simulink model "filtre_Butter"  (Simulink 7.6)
settings: Solver=ode15s  StartTime=0.0  StopTime=N  RelTol=1e-3
StopFcn:
  | courbes_butter
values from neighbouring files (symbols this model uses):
  R1 = 1e3    (= 1000)    [filtre_pbande.m]    (also in impedance_quartz.m = 30; Calcul_symbolique_RLC.m = 1)
  R2 = 100e3    (= 100000)    [_startup.m]    (also in filtre_pbande.m = 10000; Calcul_symbolique_RLC.m = 1)
libraries: fl_lib x24, nesl_utility x4, elec_lib x1

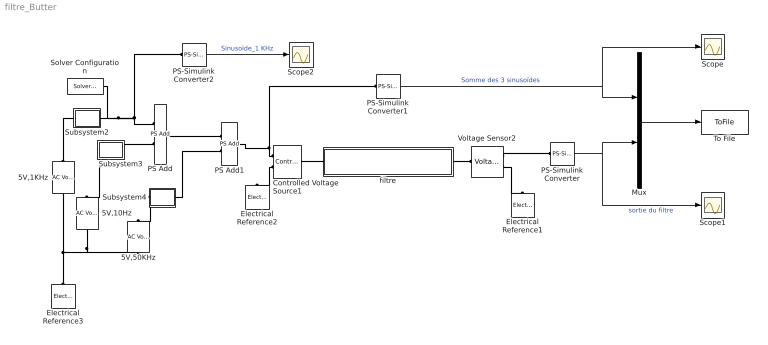
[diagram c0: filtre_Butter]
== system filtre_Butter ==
  5V,10Hz : fl_lib/Electrical/Electrical Sources/AC Voltage Source  DialogController=NetworkEngine.DynNeDlgSource  SystemSampleTime=-1  amp=5 V  shift=0 rad  omega=10 Hz  i_Log=off  v_Log=off  LocalVarNames=|current|voltage|power  LocalVarDescs=|Current (A)|Voltage (V)|Power (W)  LocalVarLogging=[0 0 0]
  5V,1KHz : fl_lib/Electrical/Electrical Sources/AC Voltage Source  DialogController=NetworkEngine.DynNeDlgSource  SystemSampleTime=-1  amp=5 V  shift=0 rad  omega=1 kHz  i_Log=off  v_Log=off  LocalVarNames=|current|voltage|power  LocalVarDescs=|Current (A)|Voltage (V)|Power (W)  LocalVarLogging=[0 0 0]
  5V,50KHz : fl_lib/Electrical/Electrical Sources/AC Voltage Source  DialogController=NetworkEngine.DynNeDlgSource  SystemSampleTime=-1  amp=5 V  shift=0 rad  omega=50 kHz  i_Log=off  v_Log=off  LocalVarNames=|current|voltage|power  LocalVarDescs=|Current (A)|Voltage (V)|Power (W)  LocalVarLogging=[0 0 0]
  Controlled Voltage Source1 : fl_lib/Electrical/Electrical Sources/Controlled Voltage Source  DialogController=NetworkEngine.DynNeDlgSource  SystemSampleTime=-1  i_Log=off  v_Log=off  LocalVarNames=|current|voltage|power  LocalVarDescs=|Current (A)|Voltage (V)|Power (W)  LocalVarLogging=[0 0 0]
  Electrical Reference1 : fl_lib/Electrical/Electrical Elements/Electrical Reference  DialogController=NetworkEngine.DynNeDlgSource  SystemSampleTime=-1  i_Log=off  LocalVarNames=|i  LocalVarDescs=|i  LocalVarLogging=0
  Electrical Reference2 : fl_lib/Electrical/Electrical Elements/Electrical Reference  DialogController=NetworkEngine.DynNeDlgSource  SystemSampleTime=-1  i_Log=off  LocalVarNames=|i  LocalVarDescs=|i  LocalVarLogging=0
  Electrical Reference3 : fl_lib/Electrical/Electrical Elements/Electrical Reference  DialogController=NetworkEngine.DynNeDlgSource  SystemSampleTime=-1  i_Log=off  LocalVarNames=|i  LocalVarDescs=|i  LocalVarLogging=0
  Mux : Mux  Inputs=2
  PS Add : fl_lib/Physical Signals/Functions/PS Add  DialogController=NetworkEngine.DynNeDlgSource  SystemSampleTime=-1  LocalVarLogging=[]
  PS Add1 : fl_lib/Physical Signals/Functions/PS Add  DialogController=NetworkEngine.DynNeDlgSource  SystemSampleTime=-1  LocalVarLogging=[]
  PS-Simulink Converter : nesl_utility/PS-Simulink Converter  DialogController=NetworkEngine.DynNeUtilDlgSource  SystemSampleTime=-1  PhysicalDomain=network_engine_domain  LeftPortType=input  RightPortType=output  SubClassName=ps_output  Unit=1  AffineConversion=off
  PS-Simulink Converter1 : nesl_utility/PS-Simulink Converter  DialogController=NetworkEngine.DynNeUtilDlgSource  SystemSampleTime=-1  PhysicalDomain=network_engine_domain  LeftPortType=input  RightPortType=output  SubClassName=ps_output  Unit=1  AffineConversion=off
  PS-Simulink Converter2 : nesl_utility/PS-Simulink Converter  DialogController=NetworkEngine.DynNeUtilDlgSource  SystemSampleTime=-1  PhysicalDomain=network_engine_domain  LeftPortType=input  RightPortType=output  SubClassName=ps_output  Unit=1  AffineConversion=off
  Scope : Scope
  Scope1 : Scope
  Scope2 : Scope
  Solver Configuration : nesl_utility/Solver Configuration  DialogController=NetworkEngine.DynNeUtilDlgSource  SystemSampleTime=-1  PhysicalDomain=network_engine_domain  LeftPortType=input  RightPortType=generic  SubClassName=solver  Accelerate=off  Profile=off  ResidualTolerance=1e-9  MaxNonlinIter=12  MaxModeIter=2  DoFixedCost=off  UseLocalSampling=off  DoDC=off  LinearAlgebra=Sparse  LocalSolverSampleTime=.001  LocalSolverChoice=NE_BACKWARD_EULER_ADVANCER  UseLocalSolver=off
  Subsystem2 : Subsystem
  Subsystem3 : Subsystem
  Subsystem4 : Subsystem
  To File : ToFile  Filename=sortie_filtre  MatrixName=s
  Voltage Sensor2 : fl_lib/Electrical/Electrical Sensors/Voltage Sensor  DialogController=NetworkEngine.DynNeDlgSource  SystemSampleTime=-1  i1_Log=off  v1_Log=off  LocalVarNames=|i1|v1  LocalVarDescs=|i1|v1  LocalVarLogging=[]
  filtre : Subsystem  InitFcn=R1=100e3;R2=100e3;C1=68e-9;C2=100e-9;N=0.001
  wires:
  PS-Simulink Converter/1 -> Mux/2, Scope1/1  "sortie du filtre"
  PS-Simulink Converter1/1 -> Mux/1, Scope/1  "Somme des 3 sinusoïdes"
  Mux/1 -> To File/1
  PS-Simulink Converter2/1 -> Scope2/1  "Sinusoïde_1 KHz"
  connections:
  Controlled Voltage Source1/LConn1 -- filtre/LConn1
  filtre/RConn1 -- Voltage Sensor2/LConn1
  Voltage Sensor2/RConn2 -- Electrical Reference1/LConn1
  Voltage Sensor2/RConn1 -- PS-Simulink Converter/LConn1
  PS Add/RConn1 -- PS Add1/LConn1
  Subsystem2/RConn1 -- Solver Configuration/RConn1 -- PS Add/LConn1 -- PS-Simulink Converter2/LConn1
  5V,1KHz/LConn1 -- Subsystem2/LConn1
  5V,50KHz/RConn1 -- 5V,10Hz/RConn1 -- 5V,1KHz/RConn1 -- Electrical Reference3/LConn1
  Subsystem3/RConn1 -- PS Add/LConn2
  Subsystem3/LConn1 -- 5V,10Hz/LConn1
  Subsystem4/LConn1 -- 5V,50KHz/LConn1
  Subsystem4/RConn1 -- PS Add1/LConn2
  Controlled Voltage Source1/RConn2 -- Electrical Reference2/LConn1
  Controlled Voltage Source1/RConn1 -- PS-Simulink Converter1/LConn1 -- PS Add1/RConn1

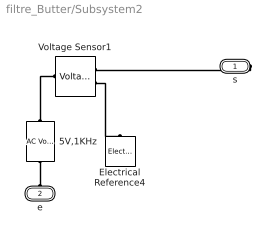
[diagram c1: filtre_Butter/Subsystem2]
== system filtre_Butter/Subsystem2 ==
  5V,1KHz : fl_lib/Electrical/Electrical Sources/AC Voltage Source  DialogController=NetworkEngine.DynNeDlgSource  SystemSampleTime=-1  amp=5 V  shift=0 rad  omega=1000 Hz  i_Log=off  v_Log=off  LocalVarNames=|current|voltage|power  LocalVarDescs=|Current (A)|Voltage (V)|Power (W)  LocalVarLogging=[0 0 0]
  Electrical Reference4 : fl_lib/Electrical/Electrical Elements/Electrical Reference  DialogController=NetworkEngine.DynNeDlgSource  SystemSampleTime=-1  i_Log=off  LocalVarNames=|i  LocalVarDescs=|i  LocalVarLogging=0
  Voltage Sensor1 : fl_lib/Electrical/Electrical Sensors/Voltage Sensor  DialogController=NetworkEngine.DynNeDlgSource  SystemSampleTime=-1  i1_Log=off  v1_Log=off  LocalVarNames=|i1|v1  LocalVarDescs=|i1|v1  LocalVarLogging=[]
  s : PMIOPort  Port=1  Side=Right
  e : PMIOPort  Port=2  Side=Left
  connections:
  5V,1KHz/LConn1 -- Voltage Sensor1/LConn1
  s/RConn1 -- Voltage Sensor1/RConn1
  e/RConn1 -- 5V,1KHz/RConn1
  Voltage Sensor1/RConn2 -- Electrical Reference4/LConn1

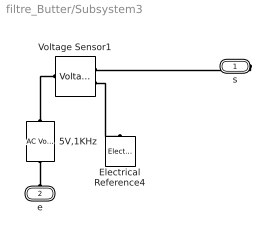
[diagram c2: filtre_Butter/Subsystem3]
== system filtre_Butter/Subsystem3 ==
  5V,1KHz : fl_lib/Electrical/Electrical Sources/AC Voltage Source  DialogController=NetworkEngine.DynNeDlgSource  SystemSampleTime=-1  amp=5 V  shift=0 rad  omega=1000 Hz  i_Log=off  v_Log=off  LocalVarNames=|current|voltage|power  LocalVarDescs=|Current (A)|Voltage (V)|Power (W)  LocalVarLogging=[0 0 0]
  Electrical Reference4 : fl_lib/Electrical/Electrical Elements/Electrical Reference  DialogController=NetworkEngine.DynNeDlgSource  SystemSampleTime=-1  i_Log=off  LocalVarNames=|i  LocalVarDescs=|i  LocalVarLogging=0
  Voltage Sensor1 : fl_lib/Electrical/Electrical Sensors/Voltage Sensor  DialogController=NetworkEngine.DynNeDlgSource  SystemSampleTime=-1  i1_Log=off  v1_Log=off  LocalVarNames=|i1|v1  LocalVarDescs=|i1|v1  LocalVarLogging=[]
  s : PMIOPort  Port=1  Side=Right
  e : PMIOPort  Port=2  Side=Left
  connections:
  Voltage Sensor1/RConn2 -- Electrical Reference4/LConn1
  e/RConn1 -- 5V,1KHz/RConn1
  s/RConn1 -- Voltage Sensor1/RConn1
  5V,1KHz/LConn1 -- Voltage Sensor1/LConn1

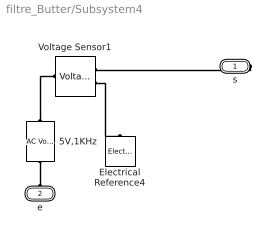
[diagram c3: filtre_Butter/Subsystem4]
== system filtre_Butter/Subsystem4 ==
  5V,1KHz : fl_lib/Electrical/Electrical Sources/AC Voltage Source  DialogController=NetworkEngine.DynNeDlgSource  SystemSampleTime=-1  amp=5 V  shift=0 rad  omega=10000 Hz  i_Log=off  v_Log=off  LocalVarNames=|current|voltage|power  LocalVarDescs=|Current (A)|Voltage (V)|Power (W)  LocalVarLogging=[0 0 0]
  Electrical Reference4 : fl_lib/Electrical/Electrical Elements/Electrical Reference  DialogController=NetworkEngine.DynNeDlgSource  SystemSampleTime=-1  i_Log=off  LocalVarNames=|i  LocalVarDescs=|i  LocalVarLogging=0
  Voltage Sensor1 : fl_lib/Electrical/Electrical Sensors/Voltage Sensor  DialogController=NetworkEngine.DynNeDlgSource  SystemSampleTime=-1  i1_Log=off  v1_Log=off  LocalVarNames=|i1|v1  LocalVarDescs=|i1|v1  LocalVarLogging=[]
  s : PMIOPort  Port=1  Side=Right
  e : PMIOPort  Port=2  Side=Left
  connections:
  5V,1KHz/LConn1 -- Voltage Sensor1/LConn1
  s/RConn1 -- Voltage Sensor1/RConn1
  e/RConn1 -- 5V,1KHz/RConn1
  Voltage Sensor1/RConn2 -- Electrical Reference4/LConn1

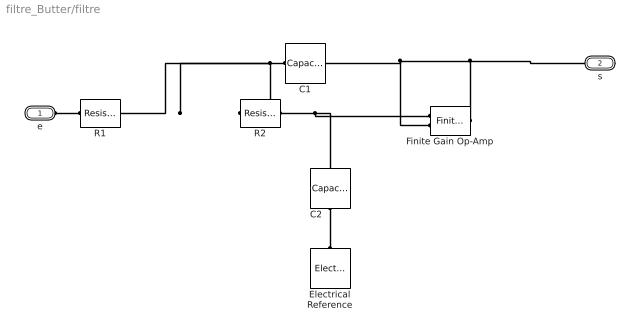
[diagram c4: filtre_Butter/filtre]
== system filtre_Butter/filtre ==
  C1 : fl_lib/Electrical/Electrical Elements/Capacitor  DialogController=NetworkEngine.DynNeDlgSource  SystemSampleTime=-1  c=C1 F  v0=0 V  r=1e-12 Ohm  g=0 1/Ohm  i_Log=off  v_Log=off  vc_Log=off  LocalVarNames=|i|v|vc  LocalVarDescs=|i|v|Internal variable for voltage across capacitor term  LocalVarLogging=[0 0 0]
  C2 : fl_lib/Electrical/Electrical Elements/Capacitor  DialogController=NetworkEngine.DynNeDlgSource  SystemSampleTime=-1  c=C2 F  v0=0 V  r=1e-12 Ohm  g=0 1/Ohm  i_Log=off  v_Log=off  vc_Log=off  LocalVarNames=|i|v|vc  LocalVarDescs=|i|v|Internal variable for voltage across capacitor term  LocalVarLogging=[0 0 0]
  Electrical Reference : fl_lib/Electrical/Electrical Elements/Electrical Reference  DialogController=NetworkEngine.DynNeDlgSource  SystemSampleTime=-1  i_Log=off  LocalVarNames=|i  LocalVarDescs=|i  LocalVarLogging=0
  Finite Gain Op-Amp : elec_lib/Integrated Circuits/Finite Gain Op-Amp  DialogController=NetworkEngine.DynNeDlgSource  SystemSampleTime=-1  A=1000  Rin=1e+6 Ohm  Rout=100 Ohm  Vmin=-15 V  Vmax=15 V  LocalVarLogging=[]
  R1 : fl_lib/Electrical/Electrical Elements/Resistor  DialogController=NetworkEngine.DynNeDlgSource  SystemSampleTime=-1  R=R1 Ohm  i_Log=off  v_Log=off  LocalVarNames=|i|v  LocalVarDescs=|i|v  LocalVarLogging=[0 0]
  R2 : fl_lib/Electrical/Electrical Elements/Resistor  DialogController=NetworkEngine.DynNeDlgSource  SystemSampleTime=-1  R=R2 Ohm  i_Log=off  v_Log=off  LocalVarNames=|i|v  LocalVarDescs=|i|v  LocalVarLogging=[0 0]
  e : PMIOPort  Port=1  Side=Left
  s : PMIOPort  Port=2  Side=Right
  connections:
  C1/LConn1 -- R1/RConn1 -- R2/LConn1
  Finite Gain Op-Amp/RConn1 -- C1/RConn1 -- Finite Gain Op-Amp/LConn2 -- s/RConn1
  C2/LConn1 -- Electrical Reference/LConn1
  e/RConn1 -- R1/LConn1
  R2/RConn1 -- Finite Gain Op-Amp/LConn1 -- C2/RConn1
